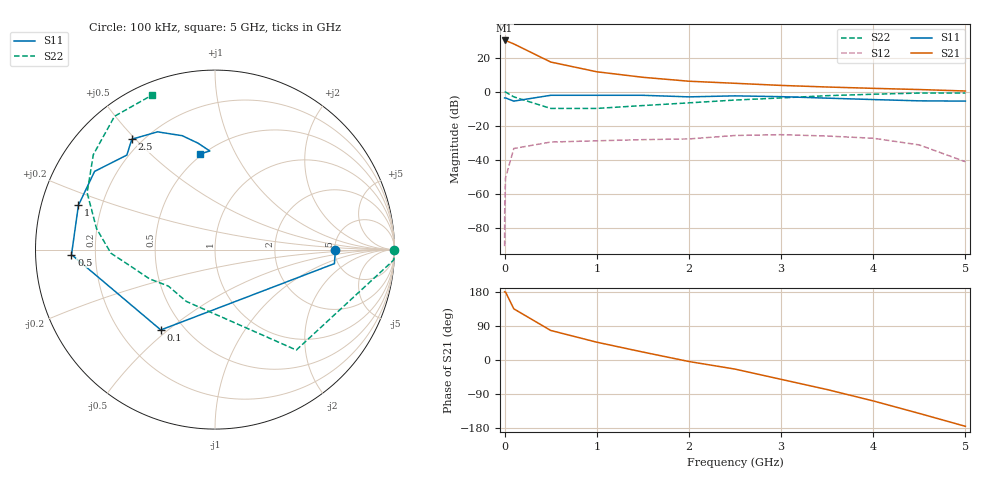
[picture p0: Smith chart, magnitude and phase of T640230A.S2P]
!AT-64023
!S-PARAMETERS at Vce=16V  Ic=110mA.  LAST UPDATED 07-21-92
# ghz s ma r 50
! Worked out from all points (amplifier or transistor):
!   14 points, 100 kHz to 5 GHz, reference 50 ohm
!   highest |S21| = 30.2 dB at 100 kHz (marker M1)
!   |S21| within 3 dB of that: start of sweep to 136.3 MHz
!   unconditionally stable (mu >= 1): 1.08 GHz to end of sweep
!   at 10 MHz: K = -0.02, MSG = 40.3 dB, |S12| = -50.5 dB
!   at 2 GHz: K = 1.89, MAG = 11.5 dB, |S12| = -27.5 dB
!   at 5 GHz: K = 5.47, MAG = 10.4 dB, |S12| = -40.9 dB
!   S11 on the Smith chart (normalised r, x): 100 kHz: 5.06, -0.02; 100 MHz: 0.37, -0.47; 500 MHz: 0.11, -0.02; 1 GHz: 0.11, +0.16; 2.5 GHz: 0.16, +0.49; 5 GHz: 0.49, +0.73
0.0001  0.67 -0.1  32.5 179.9  3e-05 88.0  0.999 0.0
0.001  0.67 -0.7  32.5 179.6  0.0003 89.0  0.999 -0.3
0.01  0.67 -6.7  32.4 179.5  0.003 87.0  0.998 -3.3
0.1  0.54 -124.0  25.71 135.0  0.022 42.0  0.72 -51.0
0.5  0.8 -178.0  7.57 78.0  0.034 18.0  0.33 -119.0
1  0.8 162.0  3.92 47.0  0.037 10.0  0.33 -142.0
1.5  0.8 147.0  2.7 21.0  0.04 12.0  0.4 -156.0
2  0.72 133.0  2.07 -4.0  0.042 1.0  0.48 -169.0
2.5  0.77 127.0  1.8 -24.0  0.053 -5.0  0.58 -178.0
3  0.73 116.0  1.56 -51.0  0.056 -20.0  0.67 170.0
3.5  0.66 106.0  1.4 -78.0  0.051 -28.0  0.78 156.0
4  0.6 99.0  1.28 -108.0  0.044 -49.0  0.86 142.0
4.5  0.55 93.0  1.18 -141.0  0.028 -70.0  0.93 127.0
5  0.54 99.0  1.07 -175.0  0.009 -144.0  0.93 112.0
